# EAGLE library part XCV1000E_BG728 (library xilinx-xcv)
xcv1000e_bg728_1532 edit this description Auto generated by make-symbol-device-package-bsdl.ulp Rev. 26 Source: xcv1000e_bg728_1532.bsd
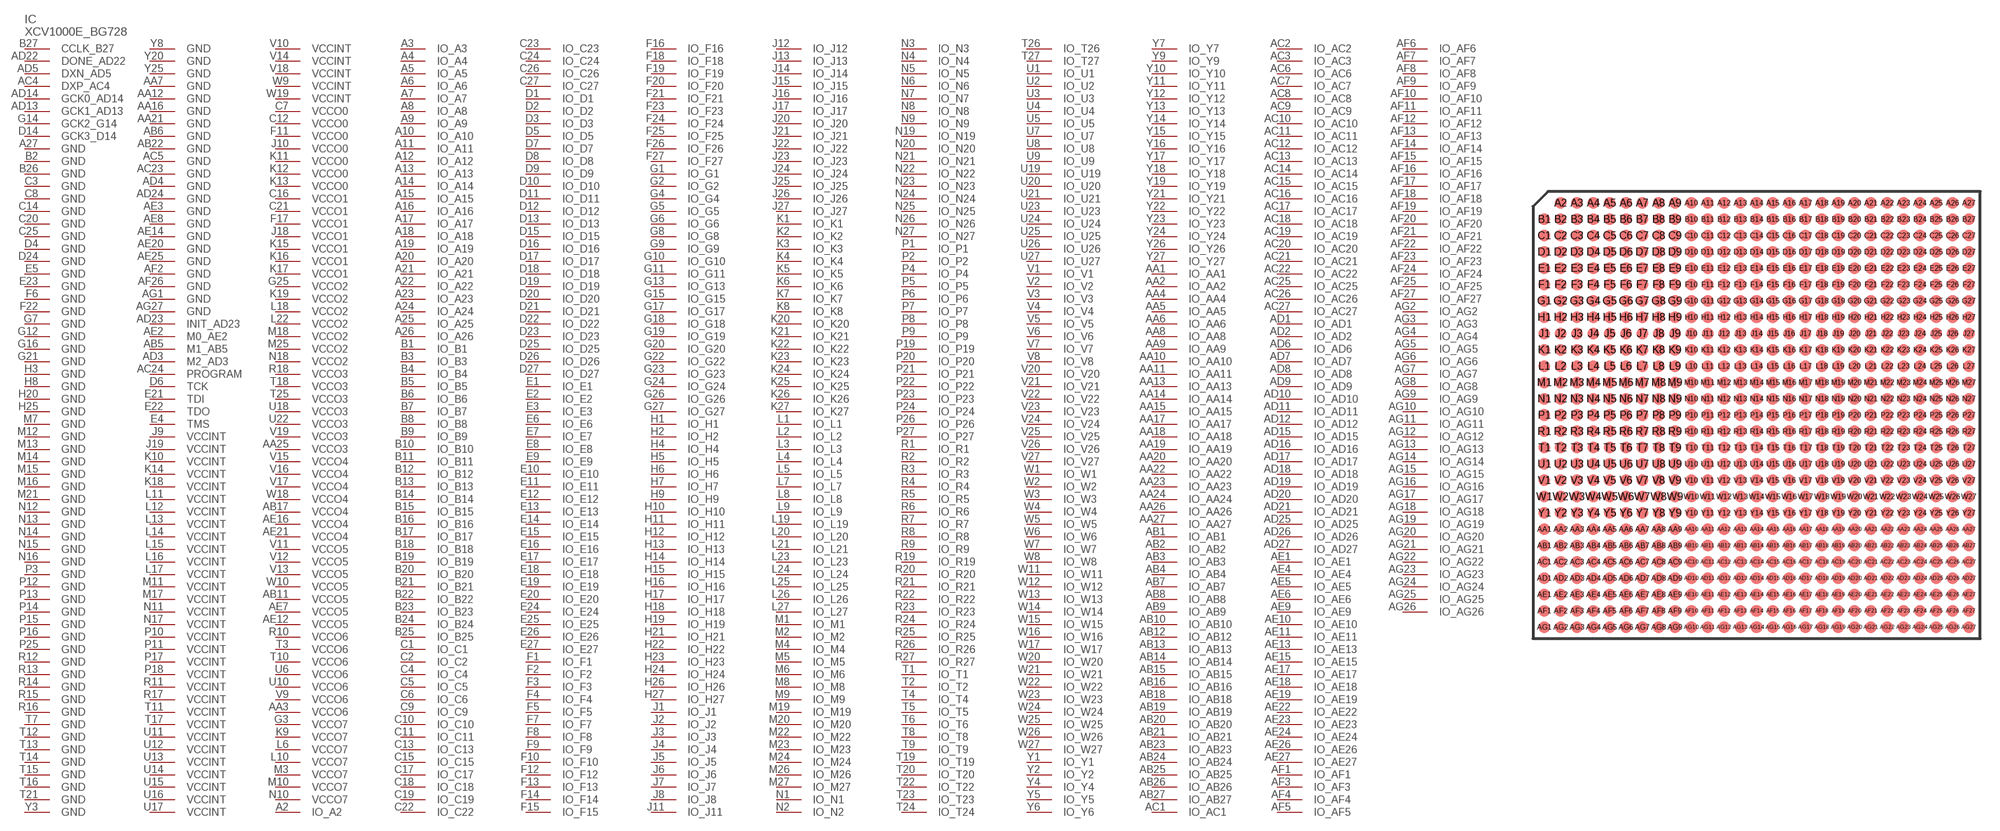
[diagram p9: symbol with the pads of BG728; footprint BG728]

Designator prefix IC

## XCV1000E_BG728 (OC_FARNELL: unknown; OC_NEWARK: unknown)  [BG728]
A2  IO_A2
A3  IO_A3
A4  IO_A4
A5  IO_A5
A6  IO_A6
A7  IO_A7
A8  IO_A8
A9  IO_A9
A10  IO_A10
A11  IO_A11
A12  IO_A12
A13  IO_A13
A14  IO_A14
A15  IO_A15
A16  IO_A16
A17  IO_A17
A18  IO_A18
A19  IO_A19
A20  IO_A20
A21  IO_A21
A22  IO_A22
A23  IO_A23
A24  IO_A24
A25  IO_A25
A26  IO_A26
A27  GND  pwr
AA1  IO_AA1
AA2  IO_AA2
AA3  VCCO6  pwr
AA4  IO_AA4
AA5  IO_AA5
AA6  IO_AA6
AA7  GND  pwr
AA8  IO_AA8
AA9  IO_AA9
AA10  IO_AA10
AA11  IO_AA11
AA12  GND  pwr
AA13  IO_AA13
AA14  IO_AA14
AA15  IO_AA15
AA16  GND  pwr
AA17  IO_AA17
AA18  IO_AA18
AA19  IO_AA19
AA20  IO_AA20
AA21  GND  pwr
AA22  IO_AA22
AA23  IO_AA23
AA24  IO_AA24
AA25  VCCO3  pwr
AA26  IO_AA26
AA27  IO_AA27
AB1  IO_AB1
AB2  IO_AB2
AB3  IO_AB3
AB4  IO_AB4
AB5  M1_AB5  in
AB6  GND  pwr
AB7  IO_AB7
AB8  IO_AB8
AB9  IO_AB9
AB10  IO_AB10
AB11  VCCO5  pwr
AB12  IO_AB12
AB13  IO_AB13
AB14  IO_AB14
AB15  IO_AB15
AB16  IO_AB16
AB17  VCCO4  pwr
AB18  IO_AB18
AB19  IO_AB19
AB20  IO_AB20
AB21  IO_AB21
AB22  GND  pwr
AB23  IO_AB23
AB24  IO_AB24
AB25  IO_AB25
AB26  IO_AB26
AB27  IO_AB27
AC1  IO_AC1
AC2  IO_AC2
AC3  IO_AC3
AC4  DXP_AC4  pas
AC5  GND  pwr
AC6  IO_AC6
AC7  IO_AC7
AC8  IO_AC8
AC9  IO_AC9
AC10  IO_AC10
AC11  IO_AC11
AC12  IO_AC12
AC13  IO_AC13
AC14  IO_AC14
AC15  IO_AC15
AC16  IO_AC16
AC17  IO_AC17
AC18  IO_AC18
AC19  IO_AC19
AC20  IO_AC20
AC21  IO_AC21
AC22  IO_AC22
AC23  GND  pwr
AC24  PROGRAM  in
AC25  IO_AC25
AC26  IO_AC26
AC27  IO_AC27
AD1  IO_AD1
AD2  IO_AD2
AD3  M2_AD3  in
AD4  GND  pwr
AD5  DXN_AD5  pas
AD6  IO_AD6
AD7  IO_AD7
AD8  IO_AD8
AD9  IO_AD9
AD10  IO_AD10
AD11  IO_AD11
AD12  IO_AD12
AD13  GCK1_AD13  in
AD14  GCK0_AD14  in
AD15  IO_AD15
AD16  IO_AD16
AD17  IO_AD17
AD18  IO_AD18
AD19  IO_AD19
AD20  IO_AD20
AD21  IO_AD21
AD22  DONE_AD22
AD23  INIT_AD23
AD24  GND  pwr
AD25  IO_AD25
AD26  IO_AD26
AD27  IO_AD27
AE1  IO_AE1
AE2  M0_AE2  in
AE3  GND  pwr
AE4  IO_AE4
AE5  IO_AE5
AE6  IO_AE6
AE7  VCCO5  pwr
AE8  GND  pwr
AE9  IO_AE9
AE10  IO_AE10
AE11  IO_AE11
AE12  VCCO5  pwr
AE13  IO_AE13
AE14  GND  pwr
AE15  IO_AE15
AE16  VCCO4  pwr
AE17  IO_AE17
AE18  IO_AE18
AE19  IO_AE19
AE20  GND  pwr
AE21  VCCO4  pwr
AE22  IO_AE22
AE23  IO_AE23
AE24  IO_AE24
AE25  GND  pwr
AE26  IO_AE26
AE27  IO_AE27
AF1  IO_AF1
AF2  GND  pwr
AF3  IO_AF3
AF4  IO_AF4
AF5  IO_AF5
AF6  IO_AF6
AF7  IO_AF7
AF8  IO_AF8
AF9  IO_AF9
AF10  IO_AF10
AF11  IO_AF11
AF12  IO_AF12
AF13  IO_AF13
AF14  IO_AF14
AF15  IO_AF15
AF16  IO_AF16
AF17  IO_AF17
AF18  IO_AF18
AF19  IO_AF19
AF20  IO_AF20
AF21  IO_AF21
AF22  IO_AF22
AF23  IO_AF23
AF24  IO_AF24
AF25  IO_AF25
AF26  GND  pwr
AF27  IO_AF27
AG1  GND  pwr
AG2  IO_AG2
AG3  IO_AG3
AG4  IO_AG4
AG5  IO_AG5
AG6  IO_AG6
AG7  IO_AG7
AG8  IO_AG8
AG9  IO_AG9
AG10  IO_AG10
AG11  IO_AG11
AG12  IO_AG12
AG13  IO_AG13
AG14  IO_AG14
AG15  IO_AG15
AG16  IO_AG16
AG17  IO_AG17
AG18  IO_AG18
AG19  IO_AG19
AG20  IO_AG20
AG21  IO_AG21
AG22  IO_AG22
AG23  IO_AG23
AG24  IO_AG24
AG25  IO_AG25
AG26  IO_AG26
AG27  GND  pwr
B1  IO_B1
B2  GND  pwr
B3  IO_B3
B4  IO_B4
B5  IO_B5
B6  IO_B6
B7  IO_B7
B8  IO_B8
B9  IO_B9
B10  IO_B10
B11  IO_B11
B12  IO_B12
B13  IO_B13
B14  IO_B14
B15  IO_B15
B16  IO_B16
B17  IO_B17
B18  IO_B18
B19  IO_B19
B20  IO_B20
B21  IO_B21
B22  IO_B22
B23  IO_B23
B24  IO_B24
B25  IO_B25
B26  GND  pwr
B27  CCLK_B27
C1  IO_C1
C2  IO_C2
C3  GND  pwr
C4  IO_C4
C5  IO_C5
C6  IO_C6
C7  VCCO0  pwr
C8  GND  pwr
C9  IO_C9
C10  IO_C10
C11  IO_C11
C12  VCCO0  pwr
C13  IO_C13
C14  GND  pwr
C15  IO_C15
C16  VCCO1  pwr
C17  IO_C17
C18  IO_C18
C19  IO_C19
C20  GND  pwr
C21  VCCO1  pwr
C22  IO_C22
C23  IO_C23
C24  IO_C24
C25  GND  pwr
C26  IO_C26
C27  IO_C27
D1  IO_D1
D2  IO_D2
D3  IO_D3
D4  GND  pwr
D5  IO_D5
D6  TCK  in
D7  IO_D7
D8  IO_D8
D9  IO_D9
D10  IO_D10
D11  IO_D11
D12  IO_D12
D13  IO_D13
D14  GCK3_D14  in
D15  IO_D15
D16  IO_D16
D17  IO_D17
D18  IO_D18
D19  IO_D19
D20  IO_D20
D21  IO_D21
D22  IO_D22
D23  IO_D23
D24  GND  pwr
D25  IO_D25
D26  IO_D26
D27  IO_D27
E1  IO_E1
E2  IO_E2
E3  IO_E3
E4  TMS  in
E5  GND  pwr
E6  IO_E6
E7  IO_E7
E8  IO_E8
E9  IO_E9
E10  IO_E10
E11  IO_E11
E12  IO_E12
E13  IO_E13
E14  IO_E14
E15  IO_E15
E16  IO_E16
E17  IO_E17
E18  IO_E18
E19  IO_E19
E20  IO_E20
E21  TDI  in
E22  TDO  out
E23  GND  pwr
E24  IO_E24
E25  IO_E25
E26  IO_E26
E27  IO_E27
F1  IO_F1
F2  IO_F2
F3  IO_F3
F4  IO_F4
F5  IO_F5
F6  GND  pwr
F7  IO_F7
F8  IO_F8
F9  IO_F9
F10  IO_F10
F11  VCCO0  pwr
F12  IO_F12
F13  IO_F13
F14  IO_F14
F15  IO_F15
F16  IO_F16
F17  VCCO1  pwr
F18  IO_F18
F19  IO_F19
F20  IO_F20
F21  IO_F21
F22  GND  pwr
F23  IO_F23
F24  IO_F24
F25  IO_F25
F26  IO_F26
F27  IO_F27
G1  IO_G1
G2  IO_G2
G3  VCCO7  pwr
G4  IO_G4
G5  IO_G5
G6  IO_G6
G7  GND  pwr
G8  IO_G8
G9  IO_G9
G10  IO_G10
G11  IO_G11
G12  GND  pwr
G13  IO_G13
G14  GCK2_G14  in
G15  IO_G15
G16  GND  pwr
G17  IO_G17
G18  IO_G18
G19  IO_G19
G20  IO_G20
G21  GND  pwr
G22  IO_G22
G23  IO_G23
G24  IO_G24
G25  VCCO2  pwr
G26  IO_G26
G27  IO_G27
H1  IO_H1
H2  IO_H2
H3  GND  pwr
H4  IO_H4
H5  IO_H5
H6  IO_H6
H7  IO_H7
H8  GND  pwr
H9  IO_H9
H10  IO_H10
H11  IO_H11
H12  IO_H12
H13  IO_H13
H14  IO_H14
H15  IO_H15
H16  IO_H16
H17  IO_H17
H18  IO_H18
H19  IO_H19
H20  GND  pwr
H21  IO_H21
H22  IO_H22
H23  IO_H23
H24  IO_H24
H25  GND  pwr
H26  IO_H26
H27  IO_H27
J1  IO_J1
J2  IO_J2
J3  IO_J3
J4  IO_J4
J5  IO_J5
J6  IO_J6
J7  IO_J7
J8  IO_J8
J9  VCCINT  pwr
J10  VCCO0  pwr
J11  IO_J11
J12  IO_J12
J13  IO_J13
J14  IO_J14
J15  IO_J15
J16  IO_J16
J17  IO_J17
J18  VCCO1  pwr
J19  VCCINT  pwr
J20  IO_J20
J21  IO_J21
J22  IO_J22
J23  IO_J23
J24  IO_J24
J25  IO_J25
J26  IO_J26
J27  IO_J27
K1  IO_K1
K2  IO_K2
K3  IO_K3
K4  IO_K4
K5  IO_K5
K6  IO_K6
K7  IO_K7
K8  IO_K8
K9  VCCO7  pwr
K10  VCCINT  pwr
K11  VCCO0  pwr
K12  VCCO0  pwr
K13  VCCO0  pwr
K14  VCCINT  pwr
K15  VCCO1  pwr
K16  VCCO1  pwr
K17  VCCO1  pwr
K18  VCCINT  pwr
K19  VCCO2  pwr
K20  IO_K20
K21  IO_K21
K22  IO_K22
K23  IO_K23
K24  IO_K24
K25  IO_K25
K26  IO_K26
K27  IO_K27
L1  IO_L1
L2  IO_L2
L3  IO_L3
L4  IO_L4
L5  IO_L5
L6  VCCO7  pwr
L7  IO_L7
L8  IO_L8
L9  IO_L9
L10  VCCO7  pwr
L11  VCCINT  pwr
L12  VCCINT  pwr
L13  VCCINT  pwr
L14  VCCINT  pwr
L15  VCCINT  pwr
L16  VCCINT  pwr
L17  VCCINT  pwr
L18  VCCO2  pwr
L19  IO_L19
L20  IO_L20
L21  IO_L21
L22  VCCO2  pwr
L23  IO_L23
L24  IO_L24
L25  IO_L25
L26  IO_L26
L27  IO_L27
M1  IO_M1
M2  IO_M2
M3  VCCO7  pwr
M4  IO_M4
M5  IO_M5
M6  IO_M6
M7  GND  pwr
M8  IO_M8
M9  IO_M9
M10  VCCO7  pwr
M11  VCCINT  pwr
M12  GND  pwr
M13  GND  pwr
M14  GND  pwr
M15  GND  pwr
M16  GND  pwr
M17  VCCINT  pwr
M18  VCCO2  pwr
M19  IO_M19
M20  IO_M20
M21  GND  pwr
M22  IO_M22
M23  IO_M23
M24  IO_M24
M25  VCCO2  pwr
M26  IO_M26
M27  IO_M27
N1  IO_N1
N2  IO_N2
N3  IO_N3
N4  IO_N4
N5  IO_N5
N6  IO_N6
N7  IO_N7
N8  IO_N8
N9  IO_N9
N10  VCCO7  pwr
N11  VCCINT  pwr
N12  GND  pwr
N13  GND  pwr
N14  GND  pwr
N15  GND  pwr
N16  GND  pwr
N17  VCCINT  pwr
N18  VCCO2  pwr
N19  IO_N19
N20  IO_N20
N21  IO_N21
N22  IO_N22
N23  IO_N23
N24  IO_N24
N25  IO_N25
N26  IO_N26
N27  IO_N27
P1  IO_P1
P2  IO_P2
P3  GND  pwr
P4  IO_P4
P5  IO_P5
P6  IO_P6
P7  IO_P7
P8  IO_P8
P9  IO_P9
P10  VCCINT  pwr
P11  VCCINT  pwr
P12  GND  pwr
P13  GND  pwr
P14  GND  pwr
P15  GND  pwr
P16  GND  pwr
P17  VCCINT  pwr
P18  VCCINT  pwr
P19  IO_P19
P20  IO_P20
P21  IO_P21
P22  IO_P22
P23  IO_P23
P24  IO_P24
P25  GND  pwr
P26  IO_P26
P27  IO_P27
R1  IO_R1
R2  IO_R2
R3  IO_R3
R4  IO_R4
R5  IO_R5
R6  IO_R6
R7  IO_R7
R8  IO_R8
R9  IO_R9
R10  VCCO6  pwr
R11  VCCINT  pwr
R12  GND  pwr
R13  GND  pwr
R14  GND  pwr
R15  GND  pwr
R16  GND  pwr
R17  VCCINT  pwr
R18  VCCO3  pwr
R19  IO_R19
R20  IO_R20
R21  IO_R21
R22  IO_R22
R23  IO_R23
R24  IO_R24
R25  IO_R25
R26  IO_R26
R27  IO_R27
T1  IO_T1
T2  IO_T2
T3  VCCO6  pwr
T4  IO_T4
T5  IO_T5
T6  IO_T6
T7  GND  pwr
T8  IO_T8
T9  IO_T9
T10  VCCO6  pwr
T11  VCCINT  pwr
T12  GND  pwr
T13  GND  pwr
T14  GND  pwr
T15  GND  pwr
T16  GND  pwr
T17  VCCINT  pwr
T18  VCCO3  pwr
T19  IO_T19
T20  IO_T20
T21  GND  pwr
T22  IO_T22
T23  IO_T23
T24  IO_T24
T25  VCCO3  pwr
T26  IO_T26
T27  IO_T27
U1  IO_U1
U2  IO_U2
U3  IO_U3
U4  IO_U4
U5  IO_U5
U6  VCCO6  pwr
U7  IO_U7
U8  IO_U8
U9  IO_U9
U10  VCCO6  pwr
U11  VCCINT  pwr
U12  VCCINT  pwr
U13  VCCINT  pwr
U14  VCCINT  pwr
U15  VCCINT  pwr
U16  VCCINT  pwr
U17  VCCINT  pwr
U18  VCCO3  pwr
U19  IO_U19
U20  IO_U20
U21  IO_U21
U22  VCCO3  pwr
U23  IO_U23
U24  IO_U24
U25  IO_U25
U26  IO_U26
U27  IO_U27
V1  IO_V1
V2  IO_V2
V3  IO_V3
V4  IO_V4
V5  IO_V5
V6  IO_V6
V7  IO_V7
V8  IO_V8
V9  VCCO6  pwr
V10  VCCINT  pwr
V11  VCCO5  pwr
V12  VCCO5  pwr
V13  VCCO5  pwr
V14  VCCINT  pwr
V15  VCCO4  pwr
V16  VCCO4  pwr
V17  VCCO4  pwr
V18  VCCINT  pwr
V19  VCCO3  pwr
V20  IO_V20
V21  IO_V21
V22  IO_V22
V23  IO_V23
V24  IO_V24
V25  IO_V25
V26  IO_V26
V27  IO_V27
W1  IO_W1
W2  IO_W2
W3  IO_W3
W4  IO_W4
W5  IO_W5
W6  IO_W6
W7  IO_W7
W8  IO_W8
W9  VCCINT  pwr
W10  VCCO5  pwr
W11  IO_W11
W12  IO_W12
W13  IO_W13
W14  IO_W14
W15  IO_W15
W16  IO_W16
W17  IO_W17
W18  VCCO4  pwr
W19  VCCINT  pwr
W20  IO_W20
W21  IO_W21
W22  IO_W22
W23  IO_W23
W24  IO_W24
W25  IO_W25
W26  IO_W26
W27  IO_W27
Y1  IO_Y1
Y2  IO_Y2
Y3  GND  pwr
Y4  IO_Y4
Y5  IO_Y5
Y6  IO_Y6
Y7  IO_Y7
Y8  GND  pwr
Y9  IO_Y9
Y10  IO_Y10
Y11  IO_Y11
Y12  IO_Y12
Y13  IO_Y13
Y14  IO_Y14
Y15  IO_Y15
Y16  IO_Y16
Y17  IO_Y17
Y18  IO_Y18
Y19  IO_Y19
Y20  GND  pwr
Y21  IO_Y21
Y22  IO_Y22
Y23  IO_Y23
Y24  IO_Y24
Y25  GND  pwr
Y26  IO_Y26
Y27  IO_Y27

## Footprint BG728 (pad centres in mm)
xcv1000e_bg728_1532 edit this description Auto generated by make-symbol-device-package-bsdl.ulp Rev. 26 Source: xcv1000e_bg728_1532.bsd
smd 0.9 x 0.9: A2 -15.24,16.51; A3 -13.97,16.51; A4 -12.7,16.51; A5 -11.43,16.51; A6 -10.16,16.51; A7 -8.89,16.51; A8 -7.62,16.51; A9 -6.35,16.51; A10 -5.08,16.51; A11 -3.81,16.51; A12 -2.54,16.51; A13 -1.27,16.51; A14 0,16.51; A15 1.27,16.51; A16 2.54,16.51; A17 3.81,16.51; A18 5.08,16.51; A19 6.35,16.51; A20 7.62,16.51; A21 8.89,16.51; A22 10.16,16.51; A23 11.43,16.51; A24 12.7,16.51; A25 13.97,16.51; A26 15.24,16.51; A27 16.51,16.51; AA1 -16.51,-8.89; AA2 -15.24,-8.89; AA3 -13.97,-8.89; AA4 -12.7,-8.89; AA5 -11.43,-8.89; AA6 -10.16,-8.89; AA7 -8.89,-8.89; AA8 -7.62,-8.89; AA9 -6.35,-8.89; AA10 -5.08,-8.89; AA11 -3.81,-8.89; AA12 -2.54,-8.89; AA13 -1.27,-8.89; AA14 0,-8.89; AA15 1.27,-8.89; AA16 2.54,-8.89; AA17 3.81,-8.89; AA18 5.08,-8.89; AA19 6.35,-8.89; AA20 7.62,-8.89; AA21 8.89,-8.89; AA22 10.16,-8.89; AA23 11.43,-8.89; AA24 12.7,-8.89; AA25 13.97,-8.89; AA26 15.24,-8.89; AA27 16.51,-8.89; AB1 -16.51,-10.16; AB2 -15.24,-10.16; AB3 -13.97,-10.16; AB4 -12.7,-10.16; AB5 -11.43,-10.16; AB6 -10.16,-10.16; AB7 -8.89,-10.16; AB8 -7.62,-10.16; AB9 -6.35,-10.16; AB10 -5.08,-10.16; AB11 -3.81,-10.16; AB12 -2.54,-10.16; AB13 -1.27,-10.16; AB14 0,-10.16; AB15 1.27,-10.16; AB16 2.54,-10.16; AB17 3.81,-10.16; AB18 5.08,-10.16; AB19 6.35,-10.16; AB20 7.62,-10.16; AB21 8.89,-10.16; AB22 10.16,-10.16; AB23 11.43,-10.16; AB24 12.7,-10.16; AB25 13.97,-10.16; AB26 15.24,-10.16; AB27 16.51,-10.16; AC1 -16.51,-11.43; AC2 -15.24,-11.43; AC3 -13.97,-11.43; AC4 -12.7,-11.43; AC5 -11.43,-11.43; AC6 -10.16,-11.43; AC7 -8.89,-11.43; AC8 -7.62,-11.43; AC9 -6.35,-11.43; AC10 -5.08,-11.43; AC11 -3.81,-11.43; AC12 -2.54,-11.43; AC13 -1.27,-11.43; AC14 0,-11.43; AC15 1.27,-11.43; AC16 2.54,-11.43; AC17 3.81,-11.43; AC18 5.08,-11.43; AC19 6.35,-11.43; AC20 7.62,-11.43; AC21 8.89,-11.43; AC22 10.16,-11.43; AC23 11.43,-11.43; AC24 12.7,-11.43; AC25 13.97,-11.43; AC26 15.24,-11.43; AC27 16.51,-11.43; AD1 -16.51,-12.7; AD2 -15.24,-12.7; AD3 -13.97,-12.7; AD4 -12.7,-12.7; AD5 -11.43,-12.7; AD6 -10.16,-12.7; AD7 -8.89,-12.7; AD8 -7.62,-12.7; AD9 -6.35,-12.7; AD10 -5.08,-12.7; AD11 -3.81,-12.7; AD12 -2.54,-12.7; AD13 -1.27,-12.7; AD14 0,-12.7; AD15 1.27,-12.7; AD16 2.54,-12.7; AD17 3.81,-12.7; AD18 5.08,-12.7; AD19 6.35,-12.7; AD20 7.62,-12.7; AD21 8.89,-12.7; AD22 10.16,-12.7; AD23 11.43,-12.7; AD24 12.7,-12.7; AD25 13.97,-12.7; AD26 15.24,-12.7; AD27 16.51,-12.7; AE1 -16.51,-13.97; AE2 -15.24,-13.97; AE3 -13.97,-13.97; AE4 -12.7,-13.97; AE5 -11.43,-13.97; AE6 -10.16,-13.97; AE7 -8.89,-13.97; AE8 -7.62,-13.97; AE9 -6.35,-13.97; AE10 -5.08,-13.97; AE11 -3.81,-13.97; AE12 -2.54,-13.97; AE13 -1.27,-13.97; AE14 0,-13.97; AE15 1.27,-13.97; AE16 2.54,-13.97; AE17 3.81,-13.97; AE18 5.08,-13.97; AE19 6.35,-13.97; AE20 7.62,-13.97; AE21 8.89,-13.97; AE22 10.16,-13.97; AE23 11.43,-13.97; AE24 12.7,-13.97; AE25 13.97,-13.97; AE26 15.24,-13.97; AE27 16.51,-13.97; AF1 -16.51,-15.24; AF2 -15.24,-15.24; AF3 -13.97,-15.24; AF4 -12.7,-15.24; AF5 -11.43,-15.24; AF6 -10.16,-15.24; AF7 -8.89,-15.24; AF8 -7.62,-15.24; AF9 -6.35,-15.24; AF10 -5.08,-15.24; AF11 -3.81,-15.24; AF12 -2.54,-15.24; AF13 -1.27,-15.24; AF14 0,-15.24; AF15 1.27,-15.24; AF16 2.54,-15.24; AF17 3.81,-15.24; AF18 5.08,-15.24; AF19 6.35,-15.24; AF20 7.62,-15.24; AF21 8.89,-15.24; AF22 10.16,-15.24; AF23 11.43,-15.24; AF24 12.7,-15.24; AF25 13.97,-15.24; AF26 15.24,-15.24; AF27 16.51,-15.24; AG1 -16.51,-16.51; AG2 -15.24,-16.51; AG3 -13.97,-16.51; AG4 -12.7,-16.51; AG5 -11.43,-16.51; AG6 -10.16,-16.51; AG7 -8.89,-16.51; AG8 -7.62,-16.51; AG9 -6.35,-16.51; AG10 -5.08,-16.51; AG11 -3.81,-16.51; AG12 -2.54,-16.51; AG13 -1.27,-16.51; AG14 0,-16.51; AG15 1.27,-16.51; AG16 2.54,-16.51; AG17 3.81,-16.51; AG18 5.08,-16.51; AG19 6.35,-16.51; AG20 7.62,-16.51; AG21 8.89,-16.51; AG22 10.16,-16.51; AG23 11.43,-16.51; AG24 12.7,-16.51; AG25 13.97,-16.51; AG26 15.24,-16.51; AG27 16.51,-16.51; B1 -16.51,15.24; B2 -15.24,15.24; B3 -13.97,15.24; B4 -12.7,15.24; B5 -11.43,15.24; B6 -10.16,15.24; B7 -8.89,15.24; B8 -7.62,15.24; B9 -6.35,15.24; B10 -5.08,15.24; B11 -3.81,15.24; B12 -2.54,15.24; B13 -1.27,15.24; B14 0,15.24; B15 1.27,15.24; B16 2.54,15.24; B17 3.81,15.24; B18 5.08,15.24; B19 6.35,15.24; B20 7.62,15.24; B21 8.89,15.24; B22 10.16,15.24; B23 11.43,15.24; B24 12.7,15.24; B25 13.97,15.24; B26 15.24,15.24; B27 16.51,15.24; C1 -16.51,13.97; C2 -15.24,13.97; C3 -13.97,13.97; C4 -12.7,13.97; C5 -11.43,13.97; C6 -10.16,13.97; C7 -8.89,13.97; C8 -7.62,13.97; C9 -6.35,13.97; C10 -5.08,13.97; C11 -3.81,13.97; C12 -2.54,13.97; C13 -1.27,13.97; C14 0,13.97; C15 1.27,13.97; C16 2.54,13.97; C17 3.81,13.97; C18 5.08,13.97; C19 6.35,13.97; C20 7.62,13.97; C21 8.89,13.97; C22 10.16,13.97; C23 11.43,13.97; C24 12.7,13.97; C25 13.97,13.97; C26 15.24,13.97; C27 16.51,13.97; D1 -16.51,12.7; D2 -15.24,12.7; D3 -13.97,12.7; D4 -12.7,12.7; D5 -11.43,12.7; D6 -10.16,12.7; D7 -8.89,12.7; D8 -7.62,12.7; D9 -6.35,12.7; D10 -5.08,12.7; D11 -3.81,12.7; D12 -2.54,12.7; D13 -1.27,12.7; D14 0,12.7; D15 1.27,12.7; D16 2.54,12.7; D17 3.81,12.7; D18 5.08,12.7; D19 6.35,12.7; D20 7.62,12.7; D21 8.89,12.7; D22 10.16,12.7; D23 11.43,12.7; D24 12.7,12.7; D25 13.97,12.7; D26 15.24,12.7; D27 16.51,12.7; E1 -16.51,11.43; E2 -15.24,11.43; E3 -13.97,11.43; E4 -12.7,11.43; E5 -11.43,11.43; E6 -10.16,11.43; E7 -8.89,11.43; E8 -7.62,11.43; E9 -6.35,11.43; E10 -5.08,11.43; E11 -3.81,11.43; E12 -2.54,11.43; E13 -1.27,11.43; E14 0,11.43; E15 1.27,11.43; E16 2.54,11.43; E17 3.81,11.43; E18 5.08,11.43; E19 6.35,11.43; E20 7.62,11.43; E21 8.89,11.43; E22 10.16,11.43; E23 11.43,11.43; E24 12.7,11.43; E25 13.97,11.43; E26 15.24,11.43; E27 16.51,11.43; F1 -16.51,10.16; F2 -15.24,10.16; F3 -13.97,10.16; F4 -12.7,10.16; F5 -11.43,10.16; F6 -10.16,10.16; F7 -8.89,10.16; F8 -7.62,10.16; F9 -6.35,10.16; F10 -5.08,10.16; F11 -3.81,10.16; F12 -2.54,10.16; F13 -1.27,10.16; F14 0,10.16; F15 1.27,10.16; F16 2.54,10.16; F17 3.81,10.16; F18 5.08,10.16; F19 6.35,10.16; F20 7.62,10.16; F21 8.89,10.16; F22 10.16,10.16; F23 11.43,10.16; F24 12.7,10.16; F25 13.97,10.16; F26 15.24,10.16; F27 16.51,10.16; G1 -16.51,8.89; G2 -15.24,8.89; G3 -13.97,8.89; G4 -12.7,8.89; G5 -11.43,8.89; G6 -10.16,8.89; G7 -8.89,8.89; G8 -7.62,8.89; G9 -6.35,8.89; G10 -5.08,8.89; G11 -3.81,8.89; G12 -2.54,8.89; G13 -1.27,8.89; G14 0,8.89; G15 1.27,8.89; G16 2.54,8.89; G17 3.81,8.89; G18 5.08,8.89; G19 6.35,8.89; G20 7.62,8.89; G21 8.89,8.89; G22 10.16,8.89; G23 11.43,8.89; G24 12.7,8.89; G25 13.97,8.89; G26 15.24,8.89; G27 16.51,8.89; H1 -16.51,7.62; H2 -15.24,7.62; H3 -13.97,7.62; H4 -12.7,7.62; H5 -11.43,7.62; H6 -10.16,7.62; H7 -8.89,7.62; H8 -7.62,7.62; H9 -6.35,7.62; H10 -5.08,7.62; H11 -3.81,7.62; H12 -2.54,7.62; H13 -1.27,7.62; H14 0,7.62; H15 1.27,7.62; H16 2.54,7.62; H17 3.81,7.62; H18 5.08,7.62; H19 6.35,7.62; H20 7.62,7.62; H21 8.89,7.62; H22 10.16,7.62; H23 11.43,7.62; H24 12.7,7.62; H25 13.97,7.62; H26 15.24,7.62; H27 16.51,7.62; J1 -16.51,6.35; J2 -15.24,6.35; J3 -13.97,6.35; J4 -12.7,6.35; J5 -11.43,6.35; J6 -10.16,6.35; J7 -8.89,6.35; J8 -7.62,6.35; J9 -6.35,6.35; J10 -5.08,6.35; J11 -3.81,6.35; J12 -2.54,6.35; J13 -1.27,6.35; J14 0,6.35; J15 1.27,6.35; J16 2.54,6.35; J17 3.81,6.35; J18 5.08,6.35; J19 6.35,6.35; J20 7.62,6.35; J21 8.89,6.35; J22 10.16,6.35; J23 11.43,6.35; J24 12.7,6.35; J25 13.97,6.35; J26 15.24,6.35; J27 16.51,6.35; K1 -16.51,5.08; K2 -15.24,5.08; K3 -13.97,5.08; K4 -12.7,5.08; K5 -11.43,5.08; K6 -10.16,5.08; K7 -8.89,5.08; K8 -7.62,5.08; K9 -6.35,5.08; K10 -5.08,5.08; K11 -3.81,5.08; K12 -2.54,5.08; K13 -1.27,5.08; K14 0,5.08; K15 1.27,5.08; K16 2.54,5.08; K17 3.81,5.08; K18 5.08,5.08; K19 6.35,5.08; K20 7.62,5.08; K21 8.89,5.08; K22 10.16,5.08; K23 11.43,5.08; K24 12.7,5.08; K25 13.97,5.08; K26 15.24,5.08; K27 16.51,5.08; L1 -16.51,3.81; L2 -15.24,3.81; L3 -13.97,3.81; L4 -12.7,3.81; L5 -11.43,3.81; L6 -10.16,3.81; L7 -8.89,3.81; L8 -7.62,3.81; L9 -6.35,3.81; L10 -5.08,3.81; L11 -3.81,3.81; L12 -2.54,3.81; L13 -1.27,3.81; L14 0,3.81; L15 1.27,3.81; L16 2.54,3.81; L17 3.81,3.81; L18 5.08,3.81; L19 6.35,3.81; L20 7.62,3.81; L21 8.89,3.81; L22 10.16,3.81; L23 11.43,3.81; L24 12.7,3.81; L25 13.97,3.81; L26 15.24,3.81; L27 16.51,3.81; M1 -16.51,2.54; M2 -15.24,2.54; M3 -13.97,2.54; M4 -12.7,2.54; M5 -11.43,2.54; M6 -10.16,2.54; M7 -8.89,2.54; M8 -7.62,2.54; M9 -6.35,2.54; M10 -5.08,2.54; M11 -3.81,2.54; M12 -2.54,2.54; M13 -1.27,2.54; M14 0,2.54; M15 1.27,2.54; M16 2.54,2.54; M17 3.81,2.54; M18 5.08,2.54; M19 6.35,2.54; M20 7.62,2.54; M21 8.89,2.54; M22 10.16,2.54; M23 11.43,2.54; M24 12.7,2.54; M25 13.97,2.54; M26 15.24,2.54; M27 16.51,2.54; N1 -16.51,1.27; N2 -15.24,1.27; N3 -13.97,1.27; N4 -12.7,1.27; N5 -11.43,1.27; N6 -10.16,1.27; N7 -8.89,1.27; N8 -7.62,1.27; N9 -6.35,1.27; N10 -5.08,1.27; N11 -3.81,1.27; N12 -2.54,1.27; N13 -1.27,1.27; N14 0,1.27; N15 1.27,1.27; N16 2.54,1.27; N17 3.81,1.27; N18 5.08,1.27; N19 6.35,1.27; N20 7.62,1.27; N21 8.89,1.27; N22 10.16,1.27; N23 11.43,1.27; N24 12.7,1.27; N25 13.97,1.27; N26 15.24,1.27; N27 16.51,1.27; P1 -16.51,0; P2 -15.24,0; P3 -13.97,0; P4 -12.7,0; P5 -11.43,0; P6 -10.16,0; P7 -8.89,0; P8 -7.62,0; P9 -6.35,0; P10 -5.08,0; P11 -3.81,0; P12 -2.54,0; P13 -1.27,0; P14 0,0; P15 1.27,0; P16 2.54,0; P17 3.81,0; P18 5.08,0; P19 6.35,0; P20 7.62,0; P21 8.89,0; P22 10.16,0; P23 11.43,0; P24 12.7,0; P25 13.97,0; P26 15.24,0; P27 16.51,0; R1 -16.51,-1.27; R2 -15.24,-1.27; R3 -13.97,-1.27; R4 -12.7,-1.27; R5 -11.43,-1.27; R6 -10.16,-1.27; R7 -8.89,-1.27; R8 -7.62,-1.27; R9 -6.35,-1.27; R10 -5.08,-1.27; R11 -3.81,-1.27; R12 -2.54,-1.27; R13 -1.27,-1.27; R14 0,-1.27; R15 1.27,-1.27; R16 2.54,-1.27; R17 3.81,-1.27; R18 5.08,-1.27; R19 6.35,-1.27; R20 7.62,-1.27; R21 8.89,-1.27; R22 10.16,-1.27; R23 11.43,-1.27; R24 12.7,-1.27; R25 13.97,-1.27; R26 15.24,-1.27; R27 16.51,-1.27; T1 -16.51,-2.54; T2 -15.24,-2.54; T3 -13.97,-2.54; T4 -12.7,-2.54; T5 -11.43,-2.54; T6 -10.16,-2.54; T7 -8.89,-2.54; T8 -7.62,-2.54; T9 -6.35,-2.54; T10 -5.08,-2.54; T11 -3.81,-2.54; T12 -2.54,-2.54; T13 -1.27,-2.54; T14 0,-2.54; T15 1.27,-2.54; T16 2.54,-2.54; T17 3.81,-2.54; T18 5.08,-2.54; T19 6.35,-2.54; T20 7.62,-2.54; T21 8.89,-2.54; T22 10.16,-2.54; T23 11.43,-2.54; T24 12.7,-2.54; T25 13.97,-2.54; T26 15.24,-2.54; T27 16.51,-2.54; U1 -16.51,-3.81; U2 -15.24,-3.81; U3 -13.97,-3.81; U4 -12.7,-3.81; U5 -11.43,-3.81; U6 -10.16,-3.81; U7 -8.89,-3.81; U8 -7.62,-3.81; U9 -6.35,-3.81; U10 -5.08,-3.81; U11 -3.81,-3.81; U12 -2.54,-3.81; U13 -1.27,-3.81; U14 0,-3.81; U15 1.27,-3.81; U16 2.54,-3.81; U17 3.81,-3.81; U18 5.08,-3.81; U19 6.35,-3.81; U20 7.62,-3.81; U21 8.89,-3.81; U22 10.16,-3.81; U23 11.43,-3.81; U24 12.7,-3.81; U25 13.97,-3.81; U26 15.24,-3.81; U27 16.51,-3.81; V1 -16.51,-5.08; V2 -15.24,-5.08; V3 -13.97,-5.08; V4 -12.7,-5.08; V5 -11.43,-5.08; V6 -10.16,-5.08; V7 -8.89,-5.08; V8 -7.62,-5.08; V9 -6.35,-5.08; V10 -5.08,-5.08; V11 -3.81,-5.08; V12 -2.54,-5.08; V13 -1.27,-5.08; V14 0,-5.08; V15 1.27,-5.08; V16 2.54,-5.08; V17 3.81,-5.08; V18 5.08,-5.08; V19 6.35,-5.08; V20 7.62,-5.08; V21 8.89,-5.08; V22 10.16,-5.08; V23 11.43,-5.08; V24 12.7,-5.08; V25 13.97,-5.08; V26 15.24,-5.08; V27 16.51,-5.08; W1 -16.51,-6.35; W2 -15.24,-6.35; W3 -13.97,-6.35; W4 -12.7,-6.35; W5 -11.43,-6.35; W6 -10.16,-6.35; W7 -8.89,-6.35; W8 -7.62,-6.35; W9 -6.35,-6.35; W10 -5.08,-6.35; W11 -3.81,-6.35; W12 -2.54,-6.35; W13 -1.27,-6.35; W14 0,-6.35; W15 1.27,-6.35; W16 2.54,-6.35; W17 3.81,-6.35; W18 5.08,-6.35; W19 6.35,-6.35; W20 7.62,-6.35; W21 8.89,-6.35; W22 10.16,-6.35; W23 11.43,-6.35; W24 12.7,-6.35; W25 13.97,-6.35; W26 15.24,-6.35; W27 16.51,-6.35; Y1 -16.51,-7.62; Y2 -15.24,-7.62; Y3 -13.97,-7.62; Y4 -12.7,-7.62; Y5 -11.43,-7.62; Y6 -10.16,-7.62; Y7 -8.89,-7.62; Y8 -7.62,-7.62; Y9 -6.35,-7.62; Y10 -5.08,-7.62; Y11 -3.81,-7.62; Y12 -2.54,-7.62; Y13 -1.27,-7.62; Y14 0,-7.62; Y15 1.27,-7.62; Y16 2.54,-7.62; Y17 3.81,-7.62; Y18 5.08,-7.62; Y19 6.35,-7.62; Y20 7.62,-7.62; Y21 8.89,-7.62; Y22 10.16,-7.62; Y23 11.43,-7.62; Y24 12.7,-7.62; Y25 13.97,-7.62; Y26 15.24,-7.62; Y27 16.51,-7.62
